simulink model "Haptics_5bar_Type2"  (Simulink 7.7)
settings: Solver=FixedStepDiscrete  SolverMode=SingleTasking  StartTime=0  StopTime=inf  FixedStep=dt  RelTol=1e-3  SampleTimeConstraint=Specified
InitFcn:
  | % Sampling Times %
  | dt0=0.001; dt1=0.1;
undefined symbols (not defined in the file or in its folder): Volts
libraries: speedgoatlib_IO311 x3, speedgoatlib x2

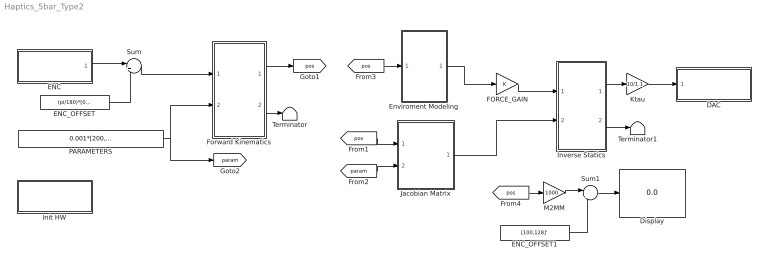
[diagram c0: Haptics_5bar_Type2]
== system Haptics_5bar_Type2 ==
  DAC : Subsystem  TreatAsAtomicUnit=on
  Display : Display
  ENC : Subsystem  TreatAsAtomicUnit=on
  ENC_OFFSET : Constant  Value=(pi/180)*[0,90]'
  ENC_OFFSET1 : Constant  Value=[100,128]'
  Enviroment Modeling : Subsystem
  FORCE_GAIN : Gain  SampleTime=dt0
  Forward Kinematics : Stateflow chart  TreatAsAtomicUnit=on
  Init HW : Subsystem  TreatAsAtomicUnit=on
  Inverse Statics : Stateflow chart  TreatAsAtomicUnit=on
  Jacobian Matrix : Stateflow chart  TreatAsAtomicUnit=on
  Ktau : Gain  Gain=10/1.1  SampleTime=dt0
  M2MM : Gain  Gain=1000  SampleTime=dt0
  PARAMETERS : Constant  Value=0.001*[200,100,100,100,100,28]
  Sum : Sum  Inputs=|++
  Sum1 : Sum  Inputs=|+-
  Terminator : Terminator
  Terminator1 : Terminator
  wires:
  Inverse Statics/1(tau) -> Ktau/1
  Inverse Statics/2(det_out) -> Terminator1/1
  FORCE_GAIN/1 -> Inverse Statics/1(force)
  ENC_OFFSET/1 -> Sum/2
  Ktau/1 -> DAC/1(In1)
  Sum/1 -> Forward Kinematics/1(th)
  PARAMETERS/1 -> Forward Kinematics/2(param), [param]
  Forward Kinematics/2(w_index) -> Terminator/1
  Forward Kinematics/1(pos) -> [pos]
  [pos] -> Jacobian Matrix/1(pos)
  [param] -> Jacobian Matrix/2(param)
  Jacobian Matrix/1(JM) -> Inverse Statics/2(JM)
  Enviroment Modeling/1(force) -> FORCE_GAIN/1
  ENC/1(Enc) -> Sum/1
  [pos] -> Enviroment Modeling/1(pos)
  [pos] -> M2MM/1
  M2MM/1 -> Sum1/1
  Sum1/1 -> Display/1
  ENC_OFFSET1/1 -> Sum1/2

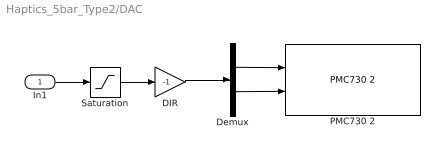
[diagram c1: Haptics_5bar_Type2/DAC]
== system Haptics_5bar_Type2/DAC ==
  In1 : Inport
  DIR : Gain  Gain=-1
  Demux : Demux  Outputs=2
  PMC730 2 : speedgoatlib/IO101/PMC730 2  id=1  channel=[1,2]  reset=[1,1]  initValue=[0,0]  ts=dt0  pciSlot=-1
  Saturation : Saturate  UpperLimit=10  LowerLimit=-10
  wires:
  In1/1 -> Saturation/1
  Saturation/1 -> DIR/1
  DIR/1 -> Demux/1
  Demux/1 -> PMC730 2/1
  Demux/2 -> PMC730 2/2

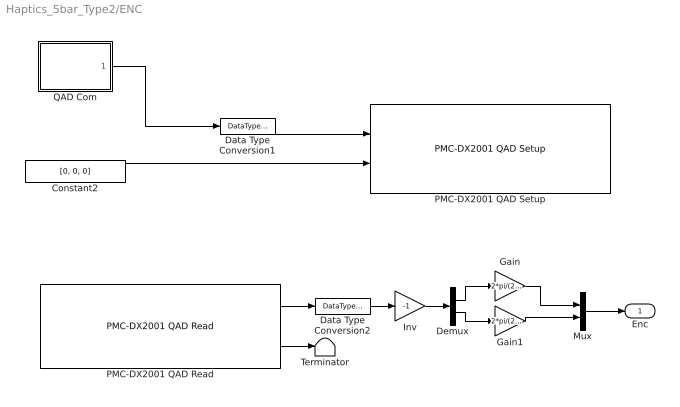
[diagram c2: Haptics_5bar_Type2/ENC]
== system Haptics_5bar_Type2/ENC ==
  Constant2 : Constant  Value=[0, 0, 0]  OutDataTypeStr=Inherit: Inherit via back propagation
  Data Type Conversion1 : DataTypeConversion  OutDataTypeStr=uint8
  Data Type Conversion2 : DataTypeConversion  OutDataTypeStr=double
  Demux : Demux  Outputs=2
  Gain : Gain  Gain=2*pi/(23*2000)
  Gain1 : Gain  Gain=2*pi/(23*2000)
  Inv : Gain  Gain=-1
  Mux : Mux  Inputs=2
  PMC-DX2001 QAD Read : speedgoatlib_IO311/PMC-DX2001 QAD Read  id=1  chan=[1, 2]  pciSlot=-1  ts=dt0
  PMC-DX2001 QAD Setup : speedgoatlib_IO311/PMC-DX2001 QAD Setup  id=1  chan=Channel 3 setup  steps1=2000  steps2=2000  steps3=2000  quadrature1=4x  quadrature2=4x  quadrature3=4x  index1=Ignore index input  index2=Ignore index input  index3=Ignore index input  special1=Disabled (cycling counter)  special2=Disabled (cycling counter)  special3=Disabled (cycling counter)  debounce=0  pciSlot=-1  ts=dt0
  QAD Com : Stateflow chart  TreatAsAtomicUnit=on
  Terminator : Terminator
  Enc : Outport
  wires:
  Constant2/1 -> PMC-DX2001 QAD Setup/2
  PMC-DX2001 QAD Read/2 -> Terminator/1
  PMC-DX2001 QAD Read/1 -> Data Type Conversion2/1
  QAD Com/1(y) -> Data Type Conversion1/1
  Data Type Conversion1/1 -> PMC-DX2001 QAD Setup/1
  Data Type Conversion2/1 -> Inv/1
  Mux/1 -> Enc/1
  Demux/1 -> Gain/1
  Gain/1 -> Mux/1
  Demux/2 -> Gain1/1
  Gain1/1 -> Mux/2
  Inv/1 -> Demux/1

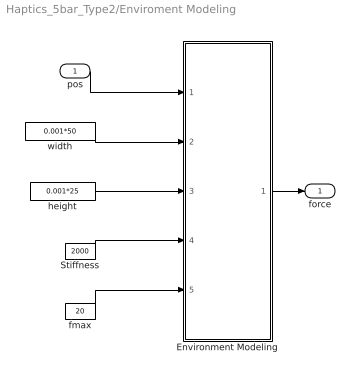
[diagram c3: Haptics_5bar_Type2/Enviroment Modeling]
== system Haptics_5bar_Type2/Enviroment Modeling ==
  pos : Inport
  Environment Modeling : Stateflow chart  TreatAsAtomicUnit=on
  Stiffness : Constant  Value=2000
  fmax : Constant  Value=20
  height : Constant  Value=0.001*25
  width : Constant  Value=0.001*50
  force : Outport
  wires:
  pos/1 -> Environment Modeling/1(pos)
  width/1 -> Environment Modeling/2(w)
  height/1 -> Environment Modeling/3(h)
  Stiffness/1 -> Environment Modeling/4(k)
  fmax/1 -> Environment Modeling/5(fmax)
  Environment Modeling/1(force) -> force/1

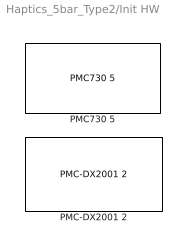
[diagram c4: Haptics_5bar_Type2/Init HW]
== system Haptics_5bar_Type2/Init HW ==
  PMC-DX2001 2 : speedgoatlib_IO311/PMC-DX2001 2  id=1  fpga1=IO311_3PWM_3CAP_3QAD_INT.fpga  fpga2=PWM_Triangle_DX501.fpga  fpga3=PWM_Triangle_DX501.fpga  fpga4=PWM_Triangle_DX501.fpga  fpga5=PWM_Triangle_DX501.fpga  fpga6=PWM_Triangle_DX501.fpga  fpga7=PWM_Triangle_DX501.fpga  fpga8=PWM_Triangle_DX501.fpga  fpga9=PWM_Triangle_DX501.fpga  fpga10=PWM_Triangle_DX501.fpga  group=Module setup  pciSlot=-1  lowerDirection=[ones(1,5), zeros(1, 7), ones(1, 1), ones(1, 3)]  lowerReset=[1]  lowerValue=[0]  upperDirection=[ones(1, 8), zeros(1, 8)]  upperReset=[1]  upperValue=[0]
  PMC730 5 : speedgoatlib/IO101/PMC730 5  id=1  group=Analog output setup  pciSlot=-1  adStartChannel=1  adNumChannel=1  adCoupling=Single-ended  adRange=-10 .. 10 Volts  adAcqMode=Standard  daChannel=[1,2]  daReset=[1,1]  daInitValue=[0,0]  diChannel=[1]  diDebounce=[0]  doChannel=[1]  doReset=[1]  doInitValue=[0]

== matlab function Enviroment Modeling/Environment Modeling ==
function force =fcn(pos, w, h, k, fmax)

px=pos(1,1)-0.1;
py=pos(2,1)-0.128;

% Check the interference along the X-axis %
def_x=0; dir_x=+1;
if px>=+w || px<=-w
    if px>=+w
        def_x=abs(px-w);
        dir_x=-1;
    end
    if px<=-w
        def_x=abs(-w-px);
        dir_x=+1;
    end        
end

% Check the interference along the Y-axis %
def_y=0; dir_y=+1;
if py>=+h || py<=-h
    if py>=+h
        def_y=abs(py-h);
        dir_y=-1;
    end
    if py<=-h
        def_y=abs(-h-py);
        dir_y=+1;
    end        
end

% f=k x dx, k=f/dx = 20N/0.010m = 2000 N/m %
fx=k*def_x; fy=k*def_y;

% fmax=20N %
if fx>=fmax, fx=fmax; end
if fy>=fmax, fy=fmax; end

force=[dir_x*fx, dir_y*fy]';

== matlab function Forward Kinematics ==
function [pos, w_index]=fcn(th, param)
persistent pos_p
if isempty(pos_p), pos_p=[100,128]'; end

L1=param(1); L2=param(2); L3=param(3); L4=param(4); L5=param(5); L6=param(6); 
th2=th(1,1); th5=th(2,1);

% (1) 
pb=[L2*cos(th2); L2*sin(th2)];
pd=[L1+L5*cos(th5); L5*sin(th5)];
% (2)
[pc, w_index]=find_intersection(pb,L3,pd,L4, +1);
if w_index==1
    % (3)
    th3=atan2(pc(2,1)-pb(2,1), pc(1,1)-pb(1,1));
    % (4)
    pos=pc+L6*[cos(th3); sin(th3)];
else
    pos=pos_p;
end
 
% Backsubstitution %
pos_p=pos;

% Find the intersection points of two circles %
function [pout, index]=find_intersection(c1,r1,c2,r2, selection)

th=atan2(c2(2,1)-c1(2,1),c2(1,1)-c1(1,1));
d=norm(c2-c1);
if d>abs(r1-r2) && d<abs(r1+r2)
    px1=(d^2+r1^2-r2^2)/(2*d);
    py1=selection*sqrt(r1^2-px1^2);
    index=1;
else
    px1=0;
    py1=0;
    index=-1;
end
pout=[cos(th)*px1-sin(th)*py1+c1(1,1);...
    sin(th)*px1+cos(th)*py1+c1(2,1)];

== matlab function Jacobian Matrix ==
function JM  =fcn(pos, param)

L1=param(1); L2=param(2); L3=param(3); L5=param(5);
%L4=param(4); L6=param(6); 

[th]=inverse_kinematics(pos, param);
th2=th(1,1); th5=th(2,1);

%pa=[0; 0];
pb=[L2*cos(th2); L2*sin(th2)];
pd=[L1+L5*cos(th5); L5*sin(th5)];
%pe=[L1;0];
th3=atan2(pos(2,1)-pb(2,1), pos(1,1)-pb(1,1));      % Absolute Angle %        
pc=pb+L3*[cos(th3); sin(th3)];
th4=atan2(pc(2,1)-pd(2,1), pc(1,1)-pd(1,1));        % Absolute Angle %

r1=L2*[cos(th2),sin(th2),0]';
r2=L5*[cos(th5),sin(th5),0]';
u1=[cos(th3),sin(th3),0]';
u2=[cos(th4),sin(th4),0]';
k=[0,0,1]';

d1=dot(cross(r1,u1),k);
d2=dot(cross(r2,u2),k);
JM=[u1(1:2,:),u2(1:2,:)]*inv(diag([d1,d2]));

%-------- Inverse Kinematics
function [th, w_index]=inverse_kinematics(pos, param)
persistent th3_p th4_p
L1=param(1); L2=param(2); L3=param(3); L4=param(4); L5=param(5); L6=param(6); 
w_index=1;
if isempty(th3_p), th3_p=0; end
if isempty(th4_p), th4_p=0; end

% (1) Left Side 2-DOF Arm %
px=pos(1,1); py=pos(2,1);
k1=(px^2+py^2-L2^2-(L3+L6)^2)/(2*L2*(L3+L6));
if abs(k1)<=1
    th3=+acos(k1);
else
    w_index=-1;
    th3=th3_p;
end

DEL1=L2^2+(L3+L6)^2+2*L2*(L3+L6)*cos(th3);
cth2=(px*(L2+(L3+L6)*cos(th3))+py*(L3+L6)*sin(th3))/DEL1;
sth2=(-px*(L3+L6)*sin(th3)+py*(L2+(L3+L6)*cos(th3)))/DEL1;
th2=atan2(sth2,cth2);

% (2) Right Side 2-DOF Arm %
cx=px-L6*cos(th2+th3)-L1; cy=py-L6*sin(th2+th3);
k2=(cx^2+cy^2-L5^2-L4^2)/(2*L5*L4);
if abs(k2)<=1
    th4=acos(k2);
else
    w_index=-2;
    th4=th4_p;
end

DEL2=L5^2+L4^2+2*L5*L4*cos(th4);
cth5=(cx*(L5+L4*cos(th4))+cy*L4*sin(th4))/DEL2;
sth5=(-cx*L4*sin(th4)+cy*(L5+L4*cos(th4)))/DEL2;
th5=atan2(sth5,cth5);

th=[th2;th5];

% Backsubstitution %
th3_p=th3; th4_p=th4;

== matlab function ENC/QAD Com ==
function y = fcn()

persistent index

if isempty(index), index=0; end

if index==0
    y=[1,1,1];      %  Reset %
else
    y = [0,0,0];
end

index=index+1;

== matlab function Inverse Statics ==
function [tau,det_out] =fcn(force, JM)

if abs(det(JM))<1.e-6
    tau=zeros(2,1);
else
    tau=inv(JM)*force;
end

[det_out]=abs(det(JM));
